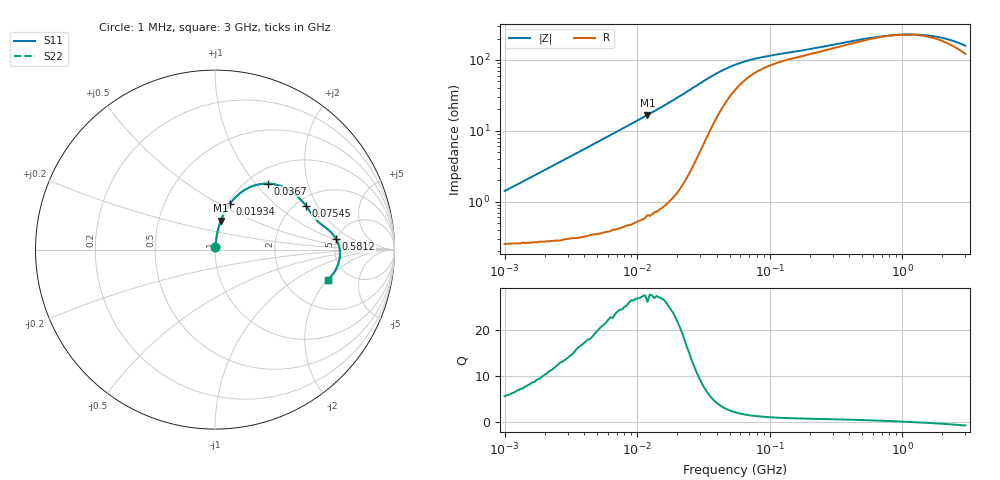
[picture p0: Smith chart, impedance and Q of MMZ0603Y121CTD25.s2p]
! S-Parameter Data Generated by TDK Corporation
! Copyright(C) 2025 TDK Corporation.
! All Rights Reserved.
! TDK P/N: MMZ0603Y121CTD25 (Chip Bead)
! Property: |Z|=120ohm at 100MHz
! Size(LxWxT): 0.6x0.3x0.3mm
! Model Type: s2p (Touchstone File Format Version 1.0)
! Frequency: DC=Yes Start=1MHz Stop=3000MHz 202points Log-sweep
! Model Generated on Feb. 6, 2025
! Terms and conditions regarding TDK Simulation Models:
! 1)This simulation model is being provided solely for informational
!  purposes. Please refer to the specifications of the products in
!  terms of detailed characteristics of such products.
! 2)In no event shall TDK Corporation of any of its subsidiaries be
!  liable for any loss or damage arising, directly or indirectly,
!  from any information contained in this simulation model, including,
!  but not limited to loss or damages arising from any inaccuracies,
!  omissions or errors in connection with such information.
! 3)Any and all copyrights on this simulation model are owned by
!  TDK Corporation.  Duplication or redistribution of this simulation
!  model without prior written permission from TDK Corporation
!  is prohibited.
! 4)This simulation model is subject to any modification or change
!  without any prior notice.
! 5)Neither TDK Corporation nor any of its subsidiaries shall make any
!  warranty, express or implied, including but not limited to the
!  correctness, implied warranties of merchantability and fitness for
!  a particular purpose with respect to this simulation models.
! 6)The use of this simulation model shall be deemed to have consented
!  to the terms and conditions hereof.
! Port Assignments:
!  1 ---@@@--- 2
! Applicable Conditions:
!  Temperature = 25 degC
!  DC Bias Current = 0 A
!  Small Signal Operation
# Hz S MA R 50
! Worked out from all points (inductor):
!   201 points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, 1 MHz to 3 GHz, reference 50 ohm
!   read as one part in series: L = 221 nH near 1.041 MHz
!   highest Q = 27.5 at 11.96 MHz (marker M1), where L = 223 nH
!   self-resonance near 1.002 GHz
!   S11 on the Smith chart (normalised r, x): 1 MHz: 1.01, +0.03; 19.34 MHz: 1.02, +0.56; 36.7 MHz: 1.23, +1.16; 75.45 MHz: 2.28, +1.61; 581.2 MHz: 4.96, +1.08; 3 GHz: 3.43, -2.04
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1000000  0.01409 78.9  0.9974 -0.8  0.9974 -0.8  0.01409 78.9
2139570  0.02961 83.0  0.9968 -1.7  0.9968 -1.7  0.02961 83.0
3900413  0.05368 83.5  0.9954 -3.1  0.9954 -3.1  0.05368 83.5
7703107  0.105 81.6  0.9902 -6.0  0.9902 -6.0  0.105 81.6
1.196486e7  0.1644 78.3  0.9801 -9.5  0.9801 -9.5  0.1644 78.3
1.461624e7  0.2004 76.3  0.9723 -11.6  0.9723 -11.6  0.2004 76.3
1.934349e7  0.2668 72.0  0.9522 -15.5  0.9522 -15.5  0.2668 72.0
2.270269e7  0.314 68.5  0.9321 -18.3  0.9321 -18.3  0.314 68.5
2.664524e7  0.3673 63.9  0.901 -21.5  0.901 -21.5  0.3673 63.9
3.127247e7  0.4221 58.1  0.8554 -24.8  0.8554 -24.8  0.4221 58.1
3.670325e7  0.4711 51.3  0.7957 -27.5  0.7957 -27.5  0.4711 51.3
4.307715e7  0.5085 44.3  0.7283 -29.2  0.7283 -29.2  0.5085 44.3
5.477226e7  0.5419 34.7  0.6348 -29.1  0.6348 -29.1  0.5419 34.7
7.544761e7  0.5628 25.4  0.5479 -26.2  0.5479 -26.2  0.5628 25.4
1.171891e8  0.5812 18.0  0.4822 -21.9  0.4822 -21.9  0.5812 18.0
2.136344e8  0.6141 12.7  0.4232 -18.6  0.4232 -18.6  0.6141 12.7
5.81181e8  0.6777 5.0  0.3302 -10.3  0.3302 -10.3  0.6777 5.0
8.005644e8  0.6896 2.1  0.3119 -4.8  0.3119 -4.8  0.6896 2.1
1.194682e9  0.6966 -1.8  0.3045 4.1  0.3045 4.1  0.6966 -1.8
1.645649e9  0.6935 -5.5  0.3168 12.1  0.3168 12.1  0.6935 -5.5
2.266846e9  0.6793 -10.1  0.352 19.8  0.352 19.8  0.6793 -10.1
3e9  0.6507 -15.3  0.4099 24.7  0.4099 24.7  0.6507 -15.3
